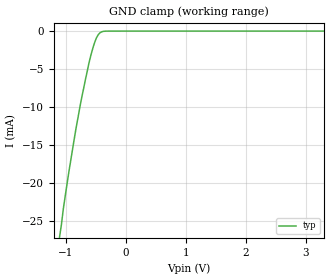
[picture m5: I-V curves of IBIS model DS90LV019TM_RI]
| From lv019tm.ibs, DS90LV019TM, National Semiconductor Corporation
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|   RECEIVER INPUT MODEL {START}
[Model]   DS90LV019TM_RI
Model_type   Input
|Signals   RIN+, RIN-
Vinh = 2.0
Vinl = 0.8
|   typ   min   max
C_comp   3.56pF   NA   NA
|   typ   min   max
[Temperature Range]   25.0   NA   NA
[Voltage range]   3.3V   3.0V   3.6V
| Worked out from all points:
|   GND clamp passes 1 mA (typ) near -0.50 V on its own axis
[GND_clamp]
|Voltage   I(typ)   I(min)   I(max)
-3.3V     -170mA     NA         NA
-1.103V   -26.98mA   NA         NA
-1.072V   -25.35mA   NA         NA
-1.041V   -23.31mA   NA         NA
-950mV    -18.54mA   NA         NA
-828mV    -12.69mA   NA         NA
-674mV    -6.399mA   NA         NA
-582mV    -3.165mA   NA         NA
-521mV    -1.531mA   NA         NA
-460mV    -479.1uA   NA         NA
-398mV    -84.39uA   NA         NA
3.3V      0A         NA         NA
[Power_clamp]
| Note that the[POWER_clamp]voltage table is referenced to Vcc
| and is calculated using Vtable=Vcc - Vmeasured.
|   Voltage   I(typ)   I(min)   I(max)
-3.3V     0A         NA         NA
0V        0A         NA         NA
